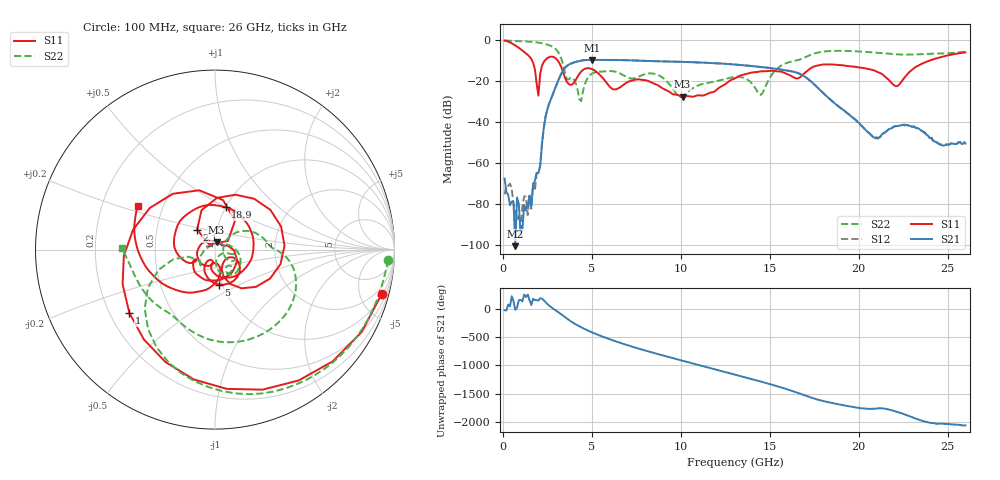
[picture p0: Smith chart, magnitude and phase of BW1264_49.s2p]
!Keysight Technologies,N5245B,MY57181159,A.13.60.06
!Date: Friday, December 18, 2020 23:54:40
!Correction: S11(Full 2 Port(1,2))
!S21(Full 2 Port(1,2))
!S12(Full 2 Port(1,2))
!S22(Full 2 Port(1,2))
!S2P File: Measurements: S11, S21, S12, S22:
# Hz S  dB  R 50
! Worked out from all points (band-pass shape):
!   260 points, 100 MHz to 26 GHz, reference 50 ohm
!   highest |S21| = -9.74 dB at 5 GHz (marker M1); lowest = -100.4 dB at 700 MHz (marker M2)
!   |S21| within 3 dB of the highest: 3.597 GHz to 14 GHz (10.41 GHz wide, 118 % of centre)
!   lowest |S11| = -27.7 dB at 10.1 GHz (marker M3), VSWR 1.09, Z = 50.7 + j4.08 ohm
!   |S11| at or under -10 dB: 1.638 GHz to 2.374 GHz (735.2 MHz wide, 36.6 % of centre); 3.08 GHz to 24.03 GHz (20.95 GHz wide, 155 % of centre)
!   |S22| runs from -29.8 to -0.3 dB; largest |S21 - S12| = 0.00054
!   S11 on the Smith chart (normalised r, x): 100 MHz: 1.15, -7.41; 1 GHz: 0.28, -0.31; 2.1 GHz: 0.80, +0.18; 5 GHz: 0.96, -0.39; 18.9 GHz: 1.00, +0.50; 26 GHz: 0.36, +0.23
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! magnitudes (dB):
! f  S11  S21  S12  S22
! 100 MHz  -0.3  -67.5  -75.3  -0.3
! 400 MHz  -1.3  -80.4  -70.0  -0.4
! 700 MHz  -2.7  -100.4  -81.7  -0.5
! 1 GHz  -4.5  -95.0  -91.5  -0.6
! 1.6 GHz  -9.3  -81.3  -82.2  -1.0
! 2 GHz  -27.2  -64.8  -64.5  -1.4
! 2.1 GHz  -16.5  -61.4  -61.2  -1.5
! 2.4 GHz  -9.7  -37.6  -37.5  -2.1
! 3 GHz  -9.2  -22.2  -22.2  -4.7
! 3.8 GHz  -21.9  -11.7  -11.7  -18.5
! 4.5 GHz  -14.7  -10.0  -10.0  -25.2
! 5 GHz  -14.2  -9.7  -9.7  -16.5
! 6.2 GHz  -24.1  -9.8  -9.8  -15.3
! 8.8 GHz  -22.6  -10.4  -10.4  -17.4
! 10.1 GHz  -27.7  -10.7  -10.7  -27.6
! 13.1 GHz  -18.5  -12.1  -12.1  -18.0
! 14.5 GHz  -15.3  -13.2  -13.2  -26.8
! 17.4 GHz  -13.3  -20.9  -20.9  -7.0
! 18.9 GHz  -12.3  -32.6  -32.6  -5.4
! 20.9 GHz  -15.0  -47.7  -47.4  -6.2
! 21.7 GHz  -19.5  -43.5  -43.5  -6.8
! 26 GHz  -6.1  -50.5  -49.7  -5.7
